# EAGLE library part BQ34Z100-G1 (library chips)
multi-chemistry wide range fuel gauge
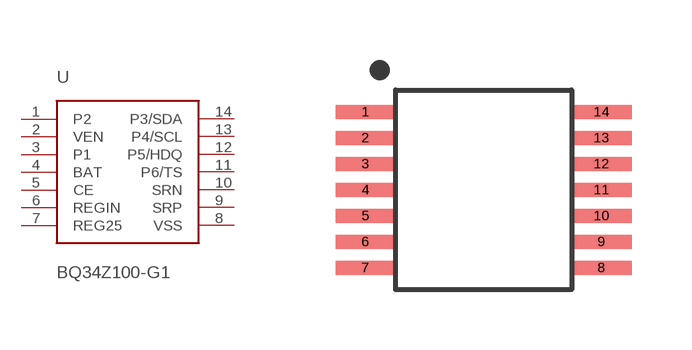
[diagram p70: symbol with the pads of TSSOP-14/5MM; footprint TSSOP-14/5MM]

Designator prefix U

## BQ34Z100-G1 (DIGIKEY: 296-39949-1-ND)  [TSSOP-14/5MM]
1  P2
2  VEN
3  P1
4  BAT
5  CE
6  REGIN
7  REG25
8  VSS
9  SRP
10  SRN
11  P6/TS
12  P5/HDQ
13  P4/SCL
14  P3/SDA

## Footprint TSSOP-14/5MM (pad centres in mm)
smd 1.5 x 0.35: 1 -2.95,1.95; 2 -2.95,1.3; 3 -2.95,0.65; 4 -2.95,0; 5 -2.95,-0.65; 6 -2.95,-1.3; 7 -2.95,-1.95; 8 2.95,-1.95; 9 2.95,-1.3; 10 2.95,-0.65; 11 2.95,0; 12 2.95,0.65; 13 2.95,1.3; 14 2.95,1.95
